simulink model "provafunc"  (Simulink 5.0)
settings: Solver=ode45  StartTime=0.0  StopTime=10.0  RelTol=1e-3
undefined symbols (not defined in the file or in its folder): inter

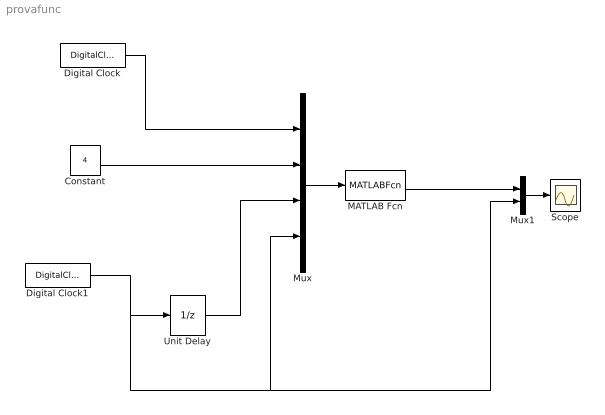
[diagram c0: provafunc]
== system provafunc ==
  Constant : Constant  Value=4  VectorParams1D=off
  Digital Clock : DigitalClock
  Digital Clock1 : DigitalClock
  MATLAB Fcn : MATLABFcn  MATLABFcn=inter(u(1),u(2),u(3),u(4))  OutputDimensions=1  OutputSignalType=real
  Mux : Mux
  Mux1 : Mux  Inputs=2
  Scope : Scope
  Unit Delay : UnitDelay
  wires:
  Digital Clock/1 -> Mux/1
  Mux/1 -> MATLAB Fcn/1
  Constant/1 -> Mux/2
  Digital Clock1/1 -> Unit Delay/1, Mux1/2, Mux/4
  MATLAB Fcn/1 -> Mux1/1
  Mux1/1 -> Scope/1
  Unit Delay/1 -> Mux/3
